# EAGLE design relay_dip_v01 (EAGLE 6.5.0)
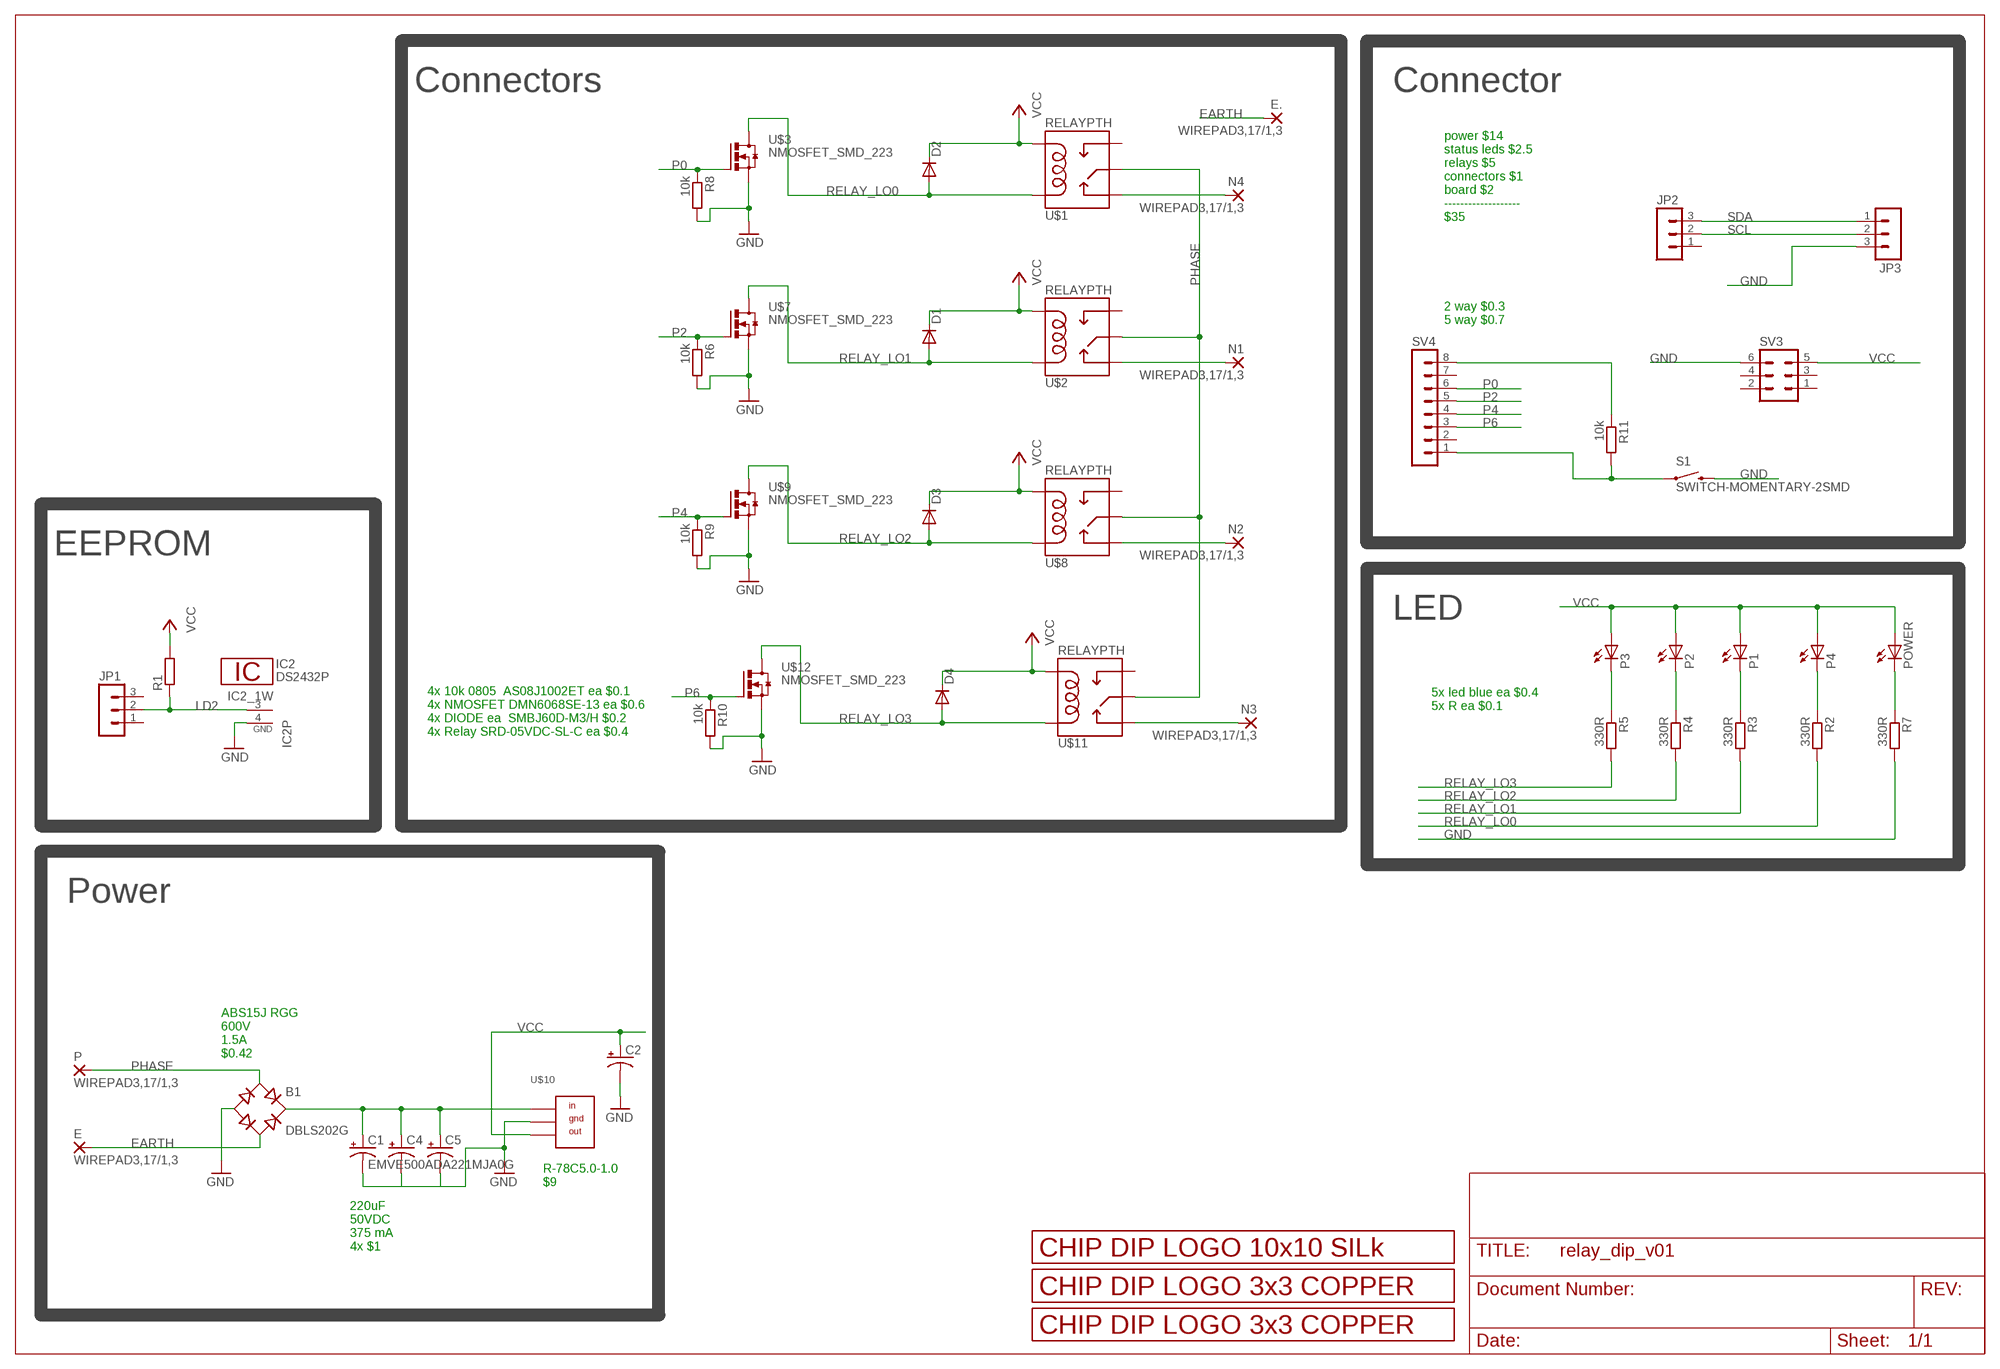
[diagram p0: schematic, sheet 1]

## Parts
B1  DBLS202G  [DBS]
C1  EMVE500ADA221MJA0G  CPOL-US150CLZ-0810  [150CLZ-0810]
C2  CPOL-US150CLZ-0810  [150CLZ-0810]
C4  CPOL-US150CLZ-0810  [150CLZ-0810]
C5  CPOL-US150CLZ-0810  [150CLZ-0810]
D1  DIODE-SMB  [SMB]
D2  DIODE-SMB  [SMB]
D3  DIODE-SMB  [SMB]
D4  DIODE-SMB  [SMB]
E  WIREPAD3,17/1,3  [3,17/1,3]
E.  WIREPAD3,17/1,3  [3,17/1,3]
IC2  DS2432P  [TSOC6]
JP1  MA03-1  [MA03-1]
JP2  MA03-1  [MA03-1]
JP3  MA03-1  [MA03-1]
N1  WIREPAD3,17/1,3  [3,17/1,3]
N2  WIREPAD3,17/1,3  [3,17/1,3]
N3  WIREPAD3,17/1,3  [3,17/1,3]
N4  WIREPAD3,17/1,3  [3,17/1,3]
P  WIREPAD3,17/1,3  [3,17/1,3]
P1  LEDCHIP-LED0805  [CHIP-LED0805]
P2  LEDCHIP-LED0805  [CHIP-LED0805]
P3  LEDCHIP-LED0805  [CHIP-LED0805]
P4  LEDCHIP-LED0805  [CHIP-LED0805]
POWER  LEDCHIP-LED0805  [CHIP-LED0805]
R1  R-EU_R0805  [R0805]
R2  330R  R-EU_R0805  [R0805]
R3  330R  R-EU_R0805  [R0805]
R4  330R  R-EU_R0805  [R0805]
R5  330R  R-EU_R0805  [R0805]
R6  10k  R-EU_R0805  [R0805]
R7  330R  R-EU_R0805  [R0805]
R8  10k  R-EU_R0805  [R0805]
R9  10k  R-EU_R0805  [R0805]
R10  10k  R-EU_R0805  [R0805]
R11  10k  R-EU_R0805  [R0805]
S1  SWITCH-MOMENTARY-2SMD  [TACTILE-SWITCH-SMD]
SV3  MA03-2  [MA03-2]
SV4  MA08-1  [MA08-1]
U$1  RELAYPTH  [SRD-05VDC-SL-C]
U$2  RELAYPTH  [SRD-05VDC-SL-C]
U$3  NMOSFET_SMD_223  [SOT223]
U$4  LOGO_3X3_COPPER  [LOGO_3X3_COPPER]
U$5  LOGO_10X10_SILK  [LOGO_10X10_SILK]
U$6  LOGO_3X3_COPPER  [LOGO_3X3_COPPER]
U$7  NMOSFET_SMD_223  [SOT223]
U$8  RELAYPTH  [SRD-05VDC-SL-C]
U$9  NMOSFET_SMD_223  [SOT223]
U$10  R-7805-1.0  [SIP3]
U$11  RELAYPTH  [SRD-05VDC-SL-C]
U$12  NMOSFET_SMD_223  [SOT223]

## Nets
EARTH: B1.AC2 E.1(P) E..1(P)
GND: B1.- C1.- C2.- C4.- C5.- IC2.4(GND) JP3.3 R6.2 R7.2 R8.2 R9.2 R10.2 S1.3 SV3.6 U$3.3(S) U$7.3(S) U$9.3(S) U$10.GND U$12.3(S)
LD2: IC2.3(1W) JP1.2 R1.1
N$1: R11.2 S1.1 SV4.1
N$3: P4.C R2.1
N$4: P1.C R3.1
N$5: B1.+ C1.+ C4.+ C5.+ U$10.IN
N$6: R11.1 SV4.8
N$8: P2.C R4.1
N$10: P3.C R5.1
N$29: POWER.C R7.1
NCL: N4.1(P) U$1.SWCLOSED(SWCLOSE)
NCL1: N1.1(P) U$2.SWCLOSED(SWCLOSE)
NCL2: N2.1(P) U$8.SWCLOSED(SWCLOSE)
NCL3: N3.1(P) U$11.SWCLOSED(SWCLOSE)
P0: R8.1 SV4.6 U$3.1(G)
P2: R6.1 SV4.5 U$7.1(G)
P4: R9.1 SV4.4 U$9.1(G)
P6: R10.1 SV4.3 U$12.1(G)
PHASE: B1.AC1 P.1(P) U$1.SWCOMMON U$2.SWCOMMON U$8.SWCOMMON U$11.SWCOMMON
RELAY_LO0: D2.A R2.2 U$1.COIL1 U$3.2(D) U$3.4(D)
RELAY_LO1: D1.A R3.2 U$2.COIL1 U$7.2(D) U$7.4(D)
RELAY_LO2: D3.A R4.2 U$8.COIL1 U$9.2(D) U$9.4(D)
RELAY_LO3: D4.A R5.2 U$11.COIL1 U$12.2(D) U$12.4(D)
SCL: JP2.2 JP3.2
SDA: JP2.3 JP3.1
VCC: C2.+ D1.C D2.C D3.C D4.C P1.A P2.A P3.A P4.A POWER.A R1.2 SV3.5 U$1.COIL0 U$2.COIL0 U$8.COIL0 U$10.OUT U$11.COIL0
Unconnected: JP1.1 JP1.3 JP2.1 SV3.1 SV3.2 SV3.3 SV3.4 SV4.2 SV4.7 U$1.SWOPEN U$2.SWOPEN U$8.SWOPEN U$11.SWOPEN

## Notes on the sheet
- Connectors | Connector
- power $14
  status leds $2.5
  relays $5
  connectors $1
  board $2
  -------------------
  $35
- 2 way $0.3
  5 way $0.7
- EEPROM
- LED
- 5x led blue ea $0.4
  5x R ea $0.1
- 4x 10k 0805  AS08J1002ET ea $0.1
  4x NMOSFET DMN6068SE-13 ea $0.6
  4x DIODE ea  SMBJ60D-M3/H $0.2
  4x Relay SRD-05VDC-SL-C ea $0.4
- Power
- ABS15J RGG
  600V
  1.5A
  $0.42
- R-78C5.0-1.0
  $9
- 220uF
  50VDC
  375 mA
  4x $1

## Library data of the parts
B1 = rectifier:DB?*G: Single Phase 1.0 AMP Glass Passivated Bridge Rectifier Taiwan Semiconductor Co.,Ltd. - TSC Source: http://www.taiwansemi.com/TSCbig5/ezcatfiles/cust/img/img/db101g.pdf http://www.ts.com.tw/db/pictures/modules/PDT/PDT060207001/DBLS201G.pdf
C1 C2 C4 C5 = rcl:CPOL-US: POLARIZED CAPACITOR, American symbol
D1-D4 = diode:DIODE-: DIODE
E E. N1-N4 P = wirepad:WIREPAD: Wire PAD connect wire on PCB
IC2 = 1wire:DS2432: 1024-Bit Protected EEPROM with SHA-1 Engine
JP1-JP3 = con-lstb:MA03-1: PIN HEADER; OC_FARNELL: unknown; OC_NEWARK: unknown
P1-P4 POWER = led:LED: LED
R1-R11 = rcl:R-EU_: RESISTOR, European symbol
S1 = SparkFun-Electromechanical:SWITCH-MOMENTARY-2: Various NO switches- pushbuttons, reed, etc; PROD_ID: SWCH-08247
SV3 = con-lstb:MA03-2: PIN HEADER; OC_FARNELL: unknown; OC_NEWARK: unknown
SV4 = con-lstb:MA08-1: PIN HEADER; OC_FARNELL: unknown; OC_NEWARK: unknown
U$1 U$2 U$8 U$11 = SRD-05VDC-SL-C:RELAY: SPDT relay (COM-00101)
U$3 U$7 U$9 U$12 = transistor-power:NMOSFET_SMD_223
U$4 U$6 = logo:LOGO_3X3_COPPER
U$5 = logo:LOGO_10X10_SILK
U$10 = Kolja:R-7805-1.0

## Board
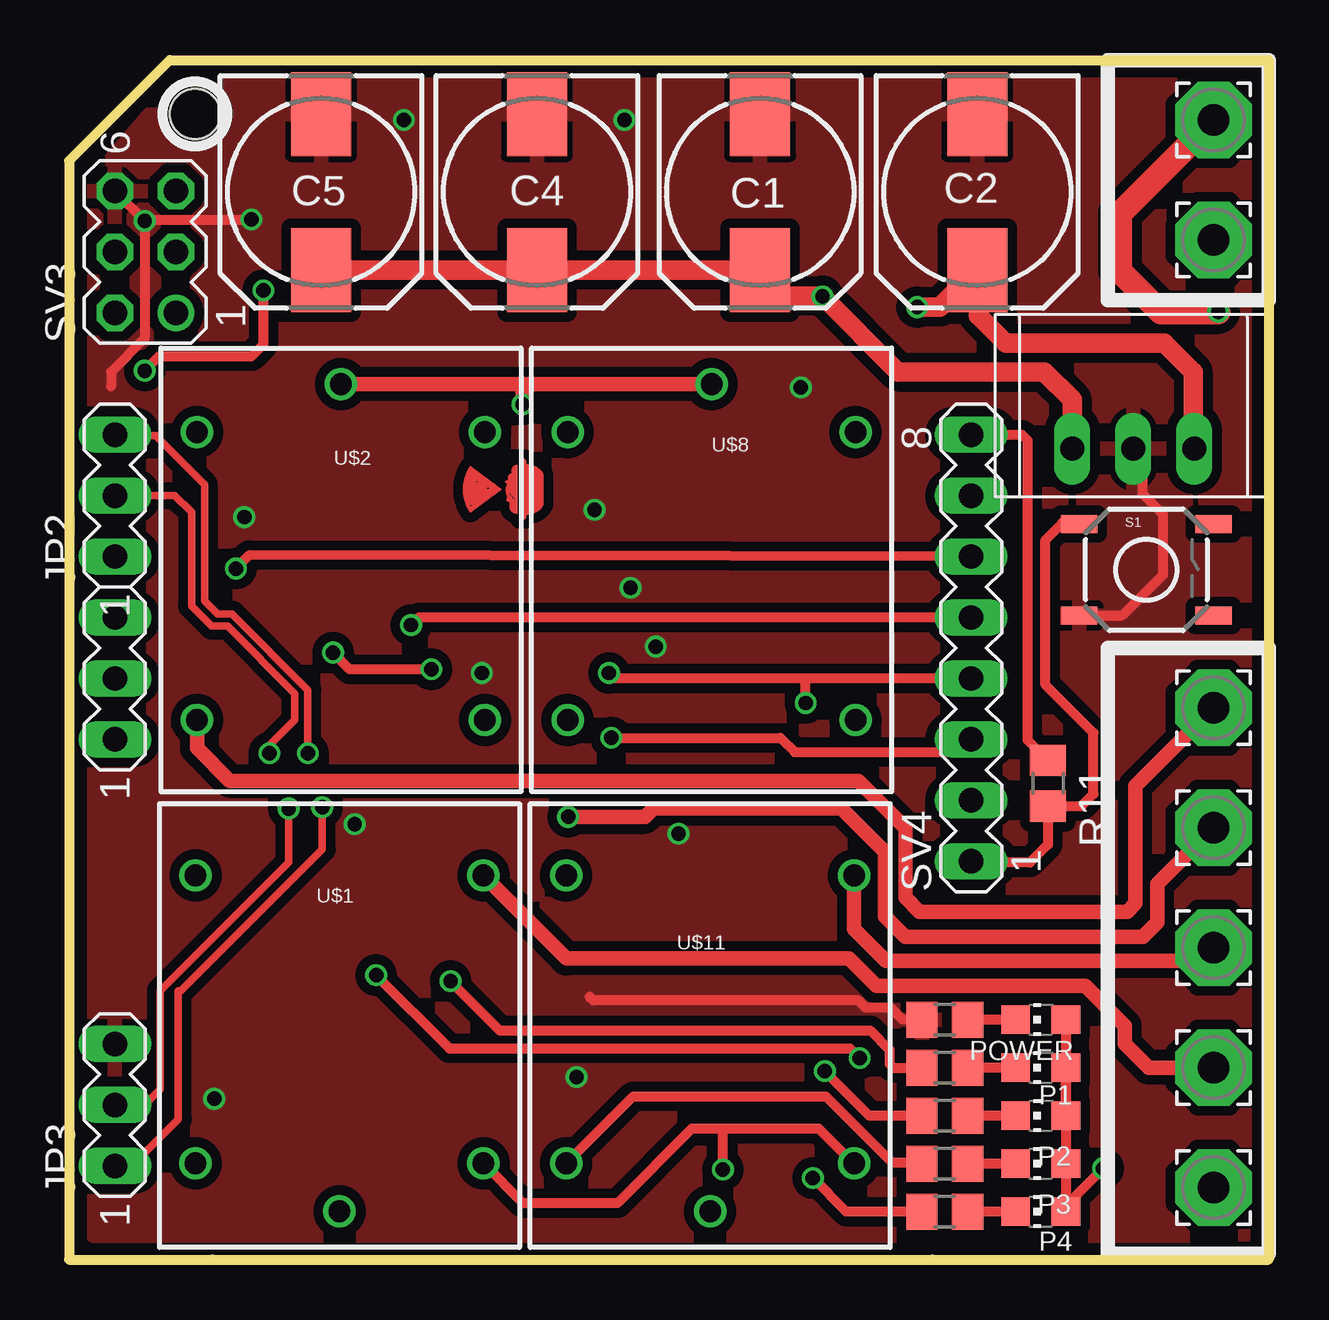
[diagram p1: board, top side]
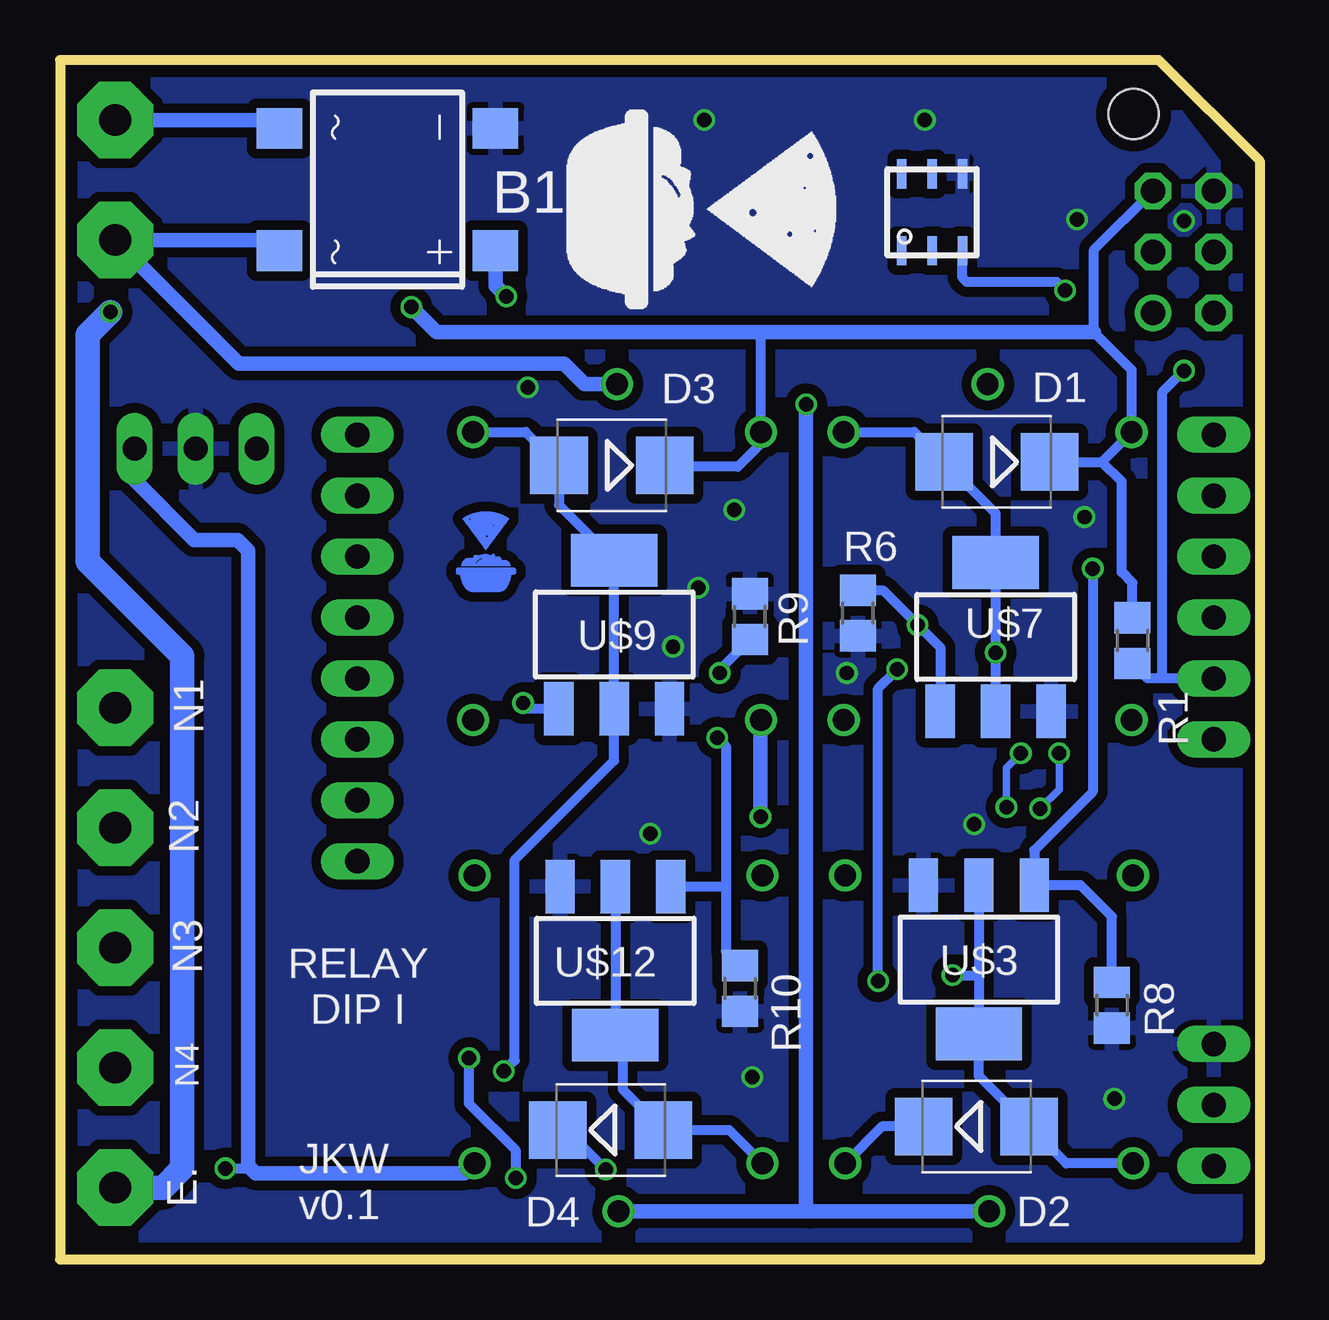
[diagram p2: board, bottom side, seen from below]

Size 50 x 50 mm. Coordinates in mm from the lower left corner, seen from the top.
Outline: 4.2,50 50,50 50,0 0,0 0,45.8 4.2,50
Copper layers (1*16): Top 0.035mm / dielectric 1.6mm / Bottom 0.035mm
Design rules "Elecrow_2-layer_PCB_eagle_rule": minimum track width 6mil, minimum drill 12mil, track to track 6mil, track to pad 6mil, pad to pad 6mil, via to via 8mil, smd to smd 0mil, copper to edge 20mil, drill to drill 10mil, minimum pad ring 6mil, minimum via ring 6mil, stop-mask expansion 0mil, vias tented up to drill 100mil, thermal gap 10mil
Holes 2.1 mm at 5.25,47.75

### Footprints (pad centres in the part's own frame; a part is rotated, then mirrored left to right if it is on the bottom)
DBS = smd 1.7 x 1.9: + -2.55,-4.5; - 2.55,-4.5; AC1 -2.55,4.5; AC2 2.55,4.5
150CLZ-0810 = smd 3.5 x 2.5: + 3.25,0; - -3.25,0
SMB = smd 2.4 x 2.4: A 2.2,0; C -2.2,0
3,17/1,3 = drill 1.321 pad 3.175 octagon: 1 0,0
TSOC6 = smd 0.406 x 1.219: 1 -1.27,-1.6; 2 0,-1.6; 3 1.27,-1.6; 4 1.27,1.6; 5 0,1.6; 6 -1.27,1.6
MA03-1 = drill 1.016 long: 1 -2.54,0; 2 0,0; 3 2.54,0
CHIP-LED0805 = smd 1.2 x 1.2: A 0,-1.05; C 0,1.05
R0805 = smd 1.3 x 1.5: 1 -0.95,0; 2 0.95,0
TACTILE-SWITCH-SMD = smd 1.524 x 0.762: 1 -2.794,1.905; 2 2.794,1.905; 3 -2.794,-1.905; 4 2.794,-1.905
MA03-2 = drill 1.016: 1 -2.54,-1.27 | drill 1.016 octagon: 2 -2.54,1.27; 3 0,-1.27; 4 0,1.27; 5 2.54,-1.27; 6 2.54,1.27
MA08-1 = drill 1.016 long: 1 -8.89,0; 2 -6.35,0; 3 -3.81,0; 4 -1.27,0; 5 1.27,0; 6 3.81,0; 7 6.35,0; 8 8.89,0
SRD-05VDC-SL-C = drill 0.9: COIL0 -5.39,-6.12; COIL1 -5.39,5.88; SWCLOSED 6.61,-6.12; SWCOMMON -7.39,-0.12; SWOPEN 6.61,5.88
SOT223 = smd 1.219 x 2.235: 1 -2.311,-3.099; 2 0,-3.099; 3 2.311,-3.099 | smd 3.6 x 2.2: 4 0,3.099
SIP3 = drill 1 long: GND 5.75,2; IN 3.21,2; OUT 8.29,2

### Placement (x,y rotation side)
B1  36.35,44.6 90 bottom
C1  28.8,44.5 270 top
C2  37.85,44.5 270 top
C4  19.5,44.5 270 top
C5  10.5,44.5 270 top
D1  10.95,33.25 180 bottom
D2  11.8,5.55 0 bottom
D3  27,33.1 180 bottom
D4  27.05,5.4 0 bottom
E  47.7,47.5 90 top
E.  47.7,3 90 top
IC2  13.65,43.65 0 bottom
JP1  1.91,24.22 90 top
JP2  1.91,31.84 90 top
JP3  1.91,6.44 90 top
N1  47.7,23 0 top
N2  47.7,18 0 top
N3  47.7,13 0 top
N4  47.7,8 90 top
P  47.7,42.5 90 top
P1  40.5,8 90 top
P2  40.5,6 90 top
P3  40.5,4 90 top
P4  40.5,2 90 top
POWER  40.5,10 90 top
R1  5.3,25.8 90 bottom
R2  36.5,2 180 top
R3  36.5,8 180 top
R4  36.5,6 180 top
R5  36.5,4 180 top
R6  16.75,26.95 270 bottom
R7  36.5,10 180 top
R8  6.15,10.6 270 bottom
R9  21.25,26.8 90 bottom
R10  21.65,11.3 270 bottom
R11  40.8,19.85 270 top
S1  44.9,28.75 0 top
SV3  3.17,42 90 top
SV4  37.6,25.49 90 top
U$1  11.15,9.4 90 top
U$2  11.45,29.1 270 top
U$3  11.7,12.5 180 bottom
U$4  18.1,32.1 90 top
U$5  28.9,47.95 270 bottom
U$6  32.25,29.5 0 bottom
U$7  11,25.95 0 bottom
U$8  26.9,29.1 270 top
U$9  26.9,26.05 0 bottom
U$10  38.6,31.8 0 top
U$11  26.6,9.4 90 top
U$12  26.85,12.45 180 bottom

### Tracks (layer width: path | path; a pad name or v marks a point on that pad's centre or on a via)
EARTH  (via drill 0.6)
  Top 1.016: E.1 43.8,43.6 43.8,41.2 45.5,39.5 v47.9,39.5
  Bottom 0.61: E.1 41.2,47.5 B1.AC2
  Bottom 1.016: E..1 45.7,3 44.9,3.8 44.9,25.15 48.85,29.1 48.85,38.55 v47.9,39.5
GND  (via drill 0.6)
  Top 0.406: v3.15,43.3 3.19,43.25 3.29,43.35 v7.6,43.35 | S1.3 43.9,26.84 45.6,28.55 45.6,31.05 44.75,31.9 44.75,33.4 U$10.GND | SV3.6 v3.15,43.3 | v3.15,43.3 3.15,38.4 1.75,37 1.75,36.4 | 21.7,10.95 21.85,10.8 32.9,10.8 33.2,10.5 34.25,10.5 34.75,10 R7.2
  other vias: 11.9,18.15 6.05,6.7 21.15,7.6 25.4,17.75 21.9,31.25 30.5,36.35 13.95,47.5 23.15,47.5 7.3,30.95 23.4,28 24.45,25.55 17.2,24.45
  pour Top (isolate 0.406): 1,1 1,45 4.4,49 49,49 49,1
  pour Bottom (isolate 0.406): 1,1 49,1 49,49 4.4,49 1,44.5
LD2  (via drill 0.6)
  Top 0.406: v3.15,37.05 3.75,37.65 7.6,37.65 8.1,38.15 v8.1,40.4
  Bottom 0.406: JP1.2 4.2,24.22 | 4.2,24.22 4.67,24.22 R1.1 | 4.2,24.22 4.05,24.37 4.05,36.15 v3.15,37.05 | v8.1,40.4 8.45,40.75 12.2,40.75 12.38,40.93 IC2.3
N$1
  Top 0.406: SV4.1 37.65,16.55 40.05,16.55 40.8,17.3 R11.2 42.2,18.9 42.7,19.4 42.7,21.95 40.7,23.95 40.7,30 41.4,30.7 42.06,30.7 S1.1
N$3
  Top 0.406: P4.C R2.1
N$4
  Top 0.406: P1.C R3.1
N$5  (via drill 0.6)
  Top 0.813: C5.+ C4.+ C1.+ 28.9,40.15 v31.4,40.15 34.55,37 40.65,37 41.81,35.84 U$10.IN
  Bottom 0.61: B1.+ 31.85,40.6 v31.4,40.15
N$6
  Top 0.406: SV4.8 39.72,34.38 39.95,34.15 39.95,21.65 R11.1
N$8
  Top 0.406: P2.C R4.1
N$10
  Top 0.406: P3.C R5.1
N$29
  Top 0.406: POWER.C R7.1
NCL
  Top 0.61: N4.1 45,8 44,9 44,9.75 42.35,11.4 33.65,11.4 32.5,12.55 20.73,12.55 U$1.SWCLOSED
NCL1
  Top 0.61: U$2.SWCLOSED 5.33,21.32 6.7,19.95 32.9,19.95 34.85,18 34.85,15.1 35.45,14.5 44.1,14.5 44.45,14.85 44.45,19.75 N1.1
NCL2  (via drill 0.6)
  Top 0.61: v20.8,18.45 24,18.45 24.35,18.8 32.2,18.8 34,17 34,14.3 34.85,13.45 44.75,13.45 45.35,14.05 45.35,15.65 N2.1
  Bottom 0.61: v20.8,18.45 20.8,22.47 U$8.SWCLOSED
NCL3
  Top 0.61: U$11.SWCLOSED 32.72,13.78 34.05,12.45 47.15,12.45 N3.1
P0  (via drill 0.6)
  Top 0.406: SV4.6 7.51,29.36 v6.95,28.8
  Bottom 0.406: v6.95,28.8 6.95,19.5 9.39,17.06 U$3.1 7.45,15.6 6.15,14.3 R8.1
P2  (via drill 0.6)
  Top 0.406: SV4.5 14.56,26.76 v14.25,26.45
  Bottom 0.406: U$7.1 13.31,25.51 v14.25,26.45 15.7,27.9 R6.1
P4  (via drill 0.6)
  Top 0.406: SV4.4 30.6,24.22 | 30.6,24.22 22.73,24.22 v22.5,24.45 | v30.7,23.2 30.7,24.12 30.6,24.22
  Bottom 0.406: v22.5,24.45 22.5,24.6 R9.1 | U$9.1 30.45,22.95 v30.7,23.2
P6  (via drill 0.6)
  Top 0.406: SV4.3 36.78,21.68 | 37.53,21.75 SV4.3 | v22.6,21.75 29.65,21.75 30.25,21.15 37.07,21.15 SV4.3
  Bottom 0.406: 22.25,15.5 22.25,21.4 v22.6,21.75 | 22.25,15.5 22.25,12.85 R10.1 | U$12.1 22.3,15.55 22.25,15.5
PHASE  (via drill 0.6)
  Top 0.61: U$8.SWCOMMON 18.9,36.49 | 18.9,36.49 U$2.SWCOMMON | v18.9,35.65 18.9,36.49
  Bottom 0.61: B1.AC1 41.3,42.5 P.1 42.55,37.35 29,37.35 28.14,36.49 U$8.SWCOMMON | U$1.SWCOMMON 18.75,2.01 | 18.75,2.01 U$11.SWCOMMON | v18.9,35.65 18.9,2.16 18.75,2.01
RELAY_LO0  (via drill 0.6)
  Top 0.406: R2.2 32.4,2 v31,3.4 | v12.8,11.85 15.85,8.8 32.55,8.8 v32.95,8.4
  Bottom 0.406: U$3.2 11.7,11.85 | 11.7,11.85 U$3.4 11.7,7.65 D2.A 8.06,4.01 U$1.COIL1 | v12.8,11.85 11.7,11.85 | v31,3.4 31,4.55 32.95,6.5 v32.95,8.4
RELAY_LO1  (via drill 0.6)
  Top 0.406: v15.1,24.6 11.7,24.6 v11,25.3 | v15.9,11.6 17.95,9.55 33.4,9.55 34.2,8.75 34.2,8.15 34.35,8 R3.2
  Bottom 0.406: U$2.COIL1 14.39,34.49 D1.A 11,31.1 U$7.4 v11,25.3 U$7.2 10.95,22.8 | v15.9,11.6 15.9,23.8 v15.1,24.6
RELAY_LO2  (via drill 0.6)
  Top 0.406: R4.2 33.35,6 v31.5,7.85
  Bottom 0.406: U$8.COIL1 30.59,34.49 D3.A 29.2,31.45 U$9.4 U$9.2 26.9,20.8 31.05,16.65 31.05,8.3 v31.5,7.85
RELAY_LO3
  Top 0.406: U$11.COIL1 23.51,6.8 31.55,6.8 34.3,4.05 35.5,4.05 R5.2
  Bottom 0.406: U$12.2 U$12.4 | U$12.4 26.85,9.2 26.55,8.9 26.55,7.1 D4.A 22.11,5.4 U$11.COIL1 | 27.2,9 U$12.4
SCL  (via drill 0.6)
  Top 0.305: JP3.2 3.15,6.45 3.8,7.1 3.8,11.2 9.15,16.55 v9.15,18.8 | JP2.2 4.41,31.84 5.1,31.15 5.1,27.25 5.95,26.4 6.6,26.4 9.4,23.6 9.4,22.5 8.35,21.45 v8.35,21.1
  Bottom 0.305: v8.35,21.1 8.35,19.6 v9.15,18.8
SDA  (via drill 0.6)
  Top 0.305: JP3.1 2.6,3.9 4.55,5.85 4.55,11.2 4.65,11.2 10.55,17.1 v10.55,18.85 | v9.95,21.1 9.95,23.75 6.8,26.9 6.2,26.9 5.65,27.45 5.65,32.3 3.6,34.35 1.94,34.35 JP2.3
  Bottom 0.305: v10.55,18.85 10.55,20.5 v9.95,21.1
VCC  (via drill 0.6)
  Top 0.406: 41.55,2.25 P2.A P1.A | 41.55,2.25 v43.1,3.8 | POWER.A P1.A | P1.A P3.A | U$11.COIL0 32.69,4.01 31.25,5.45 27.1,5.45 | 27.1,5.45 25.95,5.45 22.85,2.35 18.93,2.35 U$1.COIL0 | v27.25,3.75 27.25,5.3 27.1,5.45 | P4.A 41.55,2.25
  Top 0.813: 38.2,39.9 C2.+ | C2.+ 37.9,40.2 37.9,39.35 39.05,38.2 45.65,38.2 46.85,37 46.85,33.84 U$10.OUT | C2.+ 36.3,39.7 v35.35,39.7
  Bottom 0.406: D3.C 24.75,33.05 21.75,33.05 20.78,34.02 U$8.COIL0 20.8,34.51 20.8,38.65 | SV3.5 6.9,42.09 6.9,38.65 5.33,37.08 U$2.COIL0 6.57,33.25 | D1.C 6.57,33.25 | v43.1,3.8 42.25,3.8 42.15,3.9 | D2.C 15.73,5.55 U$1.COIL0 | D4.C 28.9,5.4 v27.25,3.75 | R1.2 5.3,28.2 5.75,28.65 5.75,32.43 6.57,33.25
  Bottom 0.61: v35.35,39.7 34.3,38.65 20.8,38.65 6.9,38.65 | U$11.COIL0 33.13,3.6 41.85,3.6 42.15,3.9 42.15,29.55 42.6,30 44.4,30 46.89,32.49 U$10.OUT

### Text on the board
bPlace: RELAY / DIP I | JKW / v0.1

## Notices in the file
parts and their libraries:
SparkFun-Electromechanical: Licensing: Creative Commons ShareAlike 4.0 International - https://creativecommons.org/licenses/by-sa/4.0
